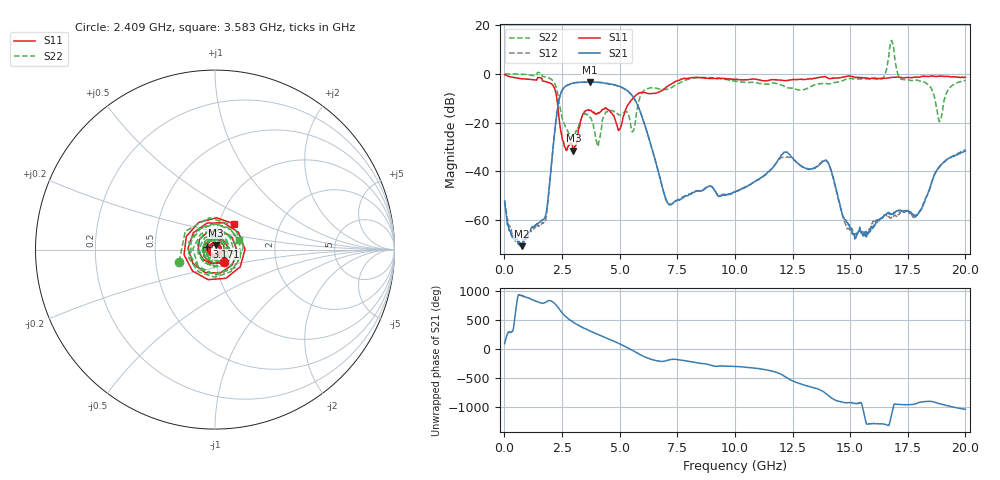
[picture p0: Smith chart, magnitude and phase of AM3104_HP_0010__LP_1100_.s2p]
!Created with skrf (http://scikit-rf.org).
# Hz S RI R 50.0
!freq ReS11 ImS11 ReS21 ImS21 ReS12 ImS12 ReS22 ImS22
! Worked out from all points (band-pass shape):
!   1601 points, 10 MHz to 20 GHz, reference 50 ohm
!   highest |S21| = -3.37 dB at 3.696 GHz (marker M1); lowest = -70.6 dB at 759.6 MHz (marker M2)
!   |S21| within 3 dB of the highest: 2.531 GHz to 5.244 GHz (2.713 GHz wide, 69.8 % of centre)
!   lowest |S11| = -31.6 dB at 2.996 GHz (marker M3), VSWR 1.05, Z = 50.5 + j2.62 ohm
!   |S11| at or under -10 dB: 2.274 GHz to 5.581 GHz (3.307 GHz wide, 84.2 % of centre)
!   |S22| runs from -29.8 to 13.6 dB; largest |S21 - S12| = 0.058
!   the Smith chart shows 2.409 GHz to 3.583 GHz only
!   S11 on the Smith chart (normalised r, x): 2.409 GHz: 1.10, -0.16; 3.171 GHz: 0.91, +0.03; 3.583 GHz: 1.18, +0.35
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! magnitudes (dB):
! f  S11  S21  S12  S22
! 10 MHz  -0.4  -52.4  -51.8  0.0
! 759.6 MHz  -2.0  -70.6  -69.3  -0.3
! 1.772 GHz  -3.2  -58.5  -60.5  -1.2
! 2.409 GHz  -21.1  -9.2  -9.2  -13.5
! 2.996 GHz  -31.6  -3.8  -3.8  -25.0
! 3.171 GHz  -26.0  -3.6  -3.6  -22.7
! 3.346 GHz  -18.2  -3.5  -3.5  -18.0
! 3.583 GHz  -15.0  -3.4  -3.5  -16.8
! 3.696 GHz  -15.1  -3.4  -3.4  -17.8
! 4.058 GHz  -16.2  -3.5  -3.5  -29.8
! 4.983 GHz  -22.9  -5.1  -5.2  -16.8
! 5.545 GHz  -10.5  -8.9  -8.9  -23.8
! 6.682 GHz  -7.6  -40.2  -40.3  -6.1
! 7.169 GHz  -4.5  -53.5  -53.8  -6.0
! 10.01 GHz  -2.4  -48.5  -48.5  -3.1
! 13.34 GHz  -2.1  -39.0  -39.1  -5.1
! 14.04 GHz  -1.8  -36.3  -36.3  -4.1
! 15.18 GHz  -1.3  -66.2  -65.9  -2.2
! 16.68 GHz  -1.6  -57.2  -58.7  7.3
! 17.9 GHz  -1.4  -57.9  -57.8  -2.7
! 18.89 GHz  -1.0  -37.9  -38.1  -19.5
! 20 GHz  -1.4  -31.7  -31.1  -2.8
